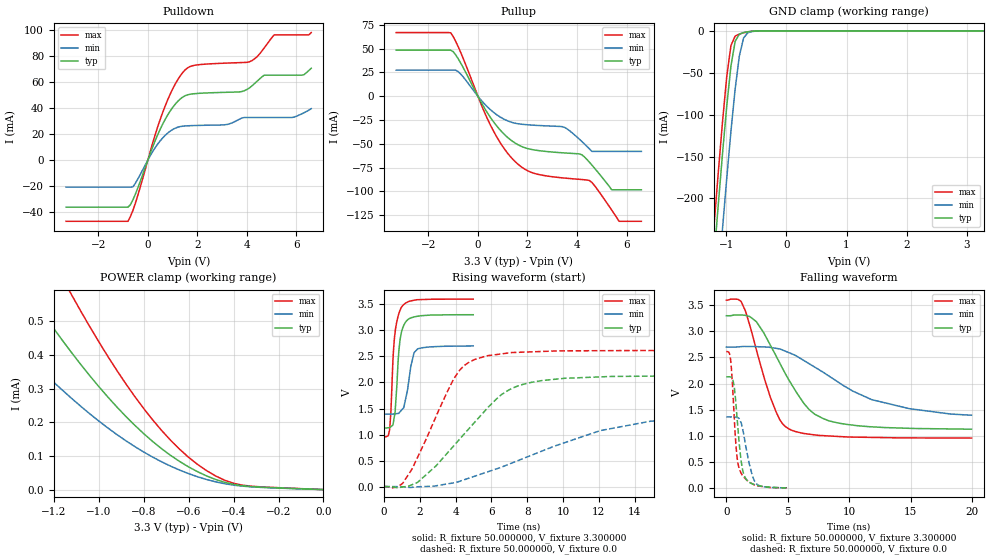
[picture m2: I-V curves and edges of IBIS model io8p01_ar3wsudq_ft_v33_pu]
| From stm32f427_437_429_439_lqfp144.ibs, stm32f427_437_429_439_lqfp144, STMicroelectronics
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|   Model io8p01_ar3wsudq_ft_v33_pu
[Model]  io8p01_ar3wsudq_ft_v33_pu
Model_type I/O
Polarity   Non-Inverting
Enable   Active-Low
Vinl =   0.990000V
Vinh =   2.310000V
Vmeas =  1.650000V
Cref =   50.000000pF
Rref =   100.000000M
Vref =   0.0V
C_comp   3.857500pF   3.760500pF   3.941700pF
[Temperature Range]   25.000000   0.125000k   -40.000000
[Pullup Reference]   3.300000V   2.700000V   3.600000V
[Pulldown Reference]   0.0V   0.0V   0.0V
[POWER Clamp Reference]   3.300000V   2.700000V   3.600000V
[GND Clamp Reference]   0.0V   0.0V   0.0V
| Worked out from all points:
|   slope of the pulldown table from 0 to 0.495 V, typ, clamps not added: 20.9 ohm
|   slope of the pullup table from 0 to 0.495 V, typ, clamps not added: 22.6 ohm
|   GND clamp passes 1 mA (typ) near -0.62 V on its own axis
|   POWER clamp passes 1 mA (typ) near -1.88 V on its own axis
|   rising waveform, R_fixture 50.000000, V_fixture 3.300000: 20-80 % time 276ps typ, 397ps min, 273ps max; typ from 1.12 V to 3.3 V
|   rising waveform, R_fixture 50.000000, V_fixture 0.0: 20-80 % time 3.36ns typ, 6.57ns min, 2.12ns max; typ from 0.001 V to 2.13 V
|   falling waveform, R_fixture 50.000000, V_fixture 3.300000: 20-80 % time 3.23ns typ, 6.16ns min, 2.04ns max; typ from 3.3 V to 1.12 V
|   falling waveform, R_fixture 50.000000, V_fixture 0.0: 20-80 % time 516ps typ, 710ps min, 443ps max; typ from 2.13 V to 0.001 V
[Pulldown]
|Voltage   I(typ)   I(min)   I(max)
-3.3V     -36.18mA   -20.77mA   -47.07mA
-800mV    -36.18mA   -20.77mA   -47.07mA
-600mV    -30.5mA    -20.52mA   -38.69mA
700mV     31.4mA     19.11mA    41.71mA
1.2V      45.15mA    25.37mA    61.75mA
1.6V      50.35mA    26.5mA     71.06mA
3.1V      52.28mA    27.26mA    74.76mA
4.1V      55.65mA    32.9mA     75.79mA
4.7V      65.5mA     32.9mA     86.49mA
5.1V      65.5mA     32.9mA     96.53mA
6.3V      65.8mA     36.47mA    96.53mA
6.6V      70.85mA    39.68mA    98.34mA
[Pullup]
|Voltage   I(typ)   I(min)   I(max)
-3.3V     48.39mA    27.39mA    66.88mA
-1.1V     48.39mA    27.39mA    66.66mA
-700mV    35.08mA    23.45mA    46.27mA
500mV     -22.06mA   -14mA      -30.03mA
1.5V      -49.1mA    -28.3mA    -68.56mA
2.2V      -56.04mA   -30.32mA   -80.35mA
3.5V      -59.52mA   -32.72mA   -85.91mA
4.2V      -61.52mA   -47.6mA    -87.45mA
4.5V      -69.2mA    -55.14mA   -88.43mA
5.4V      -98.2mA    -57.9mA    -119.4mA
5.7V      -98.2mA    -57.9mA    -131.3mA
6.6V      -98.2mA    -57.9mA    -131.3mA
[GND_clamp]
|Voltage   I(typ)   I(min)   I(max)
-3.3V     -2.333A    -2.407A    -2.313A
-1.2V     -270.2mA   -361.4mA   -232.1mA
-1.13V    -207.3mA   -298.1mA   -169mA
-1.06V    -146.7mA   -236.2mA   -108.8mA
-990mV    -90.18mA   -176.4mA   -54.96mA
-920mV    -42.21mA   -120mA     -17.68mA
-850mV    -12.57mA   -69.47mA   -6.265mA
-780mV    -3.971mA   -30.01mA   -3.886mA
-710mV    -2.1mA     -8.615mA   -2.382mA
-640mV    -1.148mA   -2.283mA   -1.22mA
-570mV    -524uA     -821.5uA   -476.8uA
3.28V     0A         0A         0A
[POWER_clamp]
|Voltage   I(typ)   I(min)   I(max)
-3.28V    1.18mA     571.5uA    1.791mA
-3.08V    1.154mA    558.1uA    1.753mA
-1.84V    973.4uA    557.7uA    1.433mA
-1.32V    593.1uA    370.2uA    831.6uA
-1.28V    553.9uA    355.9uA    778.7uA
-1.12V    406uA      270.4uA    577.3uA
-960mV    275.2uA    183.2uA    395.9uA
-800mV    166.2uA    111.7uA    240.7uA
-680mV    101.4uA    69.6uA     146.3uA
-560mV    53.02uA    38.04uA    74.62uA
-360mV    11.49uA    10.29uA    13.1uA
0V        0A         0A         0A
[Ramp]
| variable   typ   min   max
dV/dt_r  1.27741/3.36341n   0.80073/6.63752n   1.56664/2.11610n
dV/dt_f  1.30176/3.23425n   0.74178/6.20055n   1.58714/2.03718n
R_load = 50.000000
[Rising Waveform]
R_fixture= 50.000000
V_fixture= 3.300000
V_fixture_min= 2.700000
V_fixture_max= 3.600000
|time   V(typ)   V(min)   V(max)
0s        1.125V     1.393V     955.5mV
320.3ps   1.133V     1.393V     1.101V
390.4ps   1.152V     1.393V     1.458V
510.5ps   1.201V     1.393V     2.481V
650.7ps   1.58V      1.399V     3.039V
830.8ps   2.598V     1.411V     3.319V
991ps     2.982V     1.472V     3.451V
1.682ns   3.257V     2.571V     3.577V
1.882ns   3.271V     2.644V     3.588V
4.985ns   3.3V       2.7V       3.599V
[Rising Waveform]
R_fixture= 50.000000
V_fixture= 0.0
V_fixture_min= 0.0
V_fixture_max= 0.0
|time   V(typ)   V(min)   V(max)
0s        1.284mV    1.126mV    1.857mV
1.041ns   -6.608mV   -3.2mV     61.37mV
1.882ns   83.11mV    -2.203mV   566.5mV
3.844ns   763.4mV    70.41mV    2.034V
5.045ns   1.228V     198mV      2.438V
6.607ns   1.777V     380.8mV    2.55V
8.208ns   2V         599.3mV    2.587V
12.09ns   2.107V     1.077V     2.61V
14.89ns   2.121V     1.256V     2.612V
19.94ns   2.129V     1.36V      2.612V
[Falling Waveform]
R_fixture= 50.000000
V_fixture= 3.300000
V_fixture_min= 2.700000
V_fixture_max= 3.600000
|time   V(typ)   V(min)   V(max)
0s        3.3V       2.7V       3.599V
1.201ns   3.314V     2.708V     3.574V
2.442ns   3.186V     2.707V     2.648V
3.604ns   2.726V     2.691V     1.724V
4.364ns   2.384V     2.662V     1.301V
5.085ns   2.069V     2.592V     1.132V
6.727ns   1.503V     2.381V     1.03V
8.328ns   1.287V     2.146V     996mV
11.85ns   1.17V      1.69V      967.8mV
19.94ns   1.125V     1.393V     955.5mV
[Falling Waveform]
R_fixture= 50.000000
V_fixture= 0.0
V_fixture_min= 0.0
V_fixture_max= 0.0
|time   V(typ)   V(min)   V(max)
0s        2.129V     1.36V      2.612V
340.3ps   2.126V     1.359V     2.474V
500.5ps   2.083V     1.359V     1.969V
640.6ps   1.941V     1.359V     1.361V
880.9ps   1.322V     1.349V     573.3mV
1.171ns   578.9mV    1.263V     297mV
1.512ns   206.7mV    894.1mV    183.9mV
1.852ns   109.9mV    473.5mV    113.3mV
2.312ns   61.56mV    121.9mV    53.82mV
4.985ns   1.284mV    1.126mV    1.857mV
